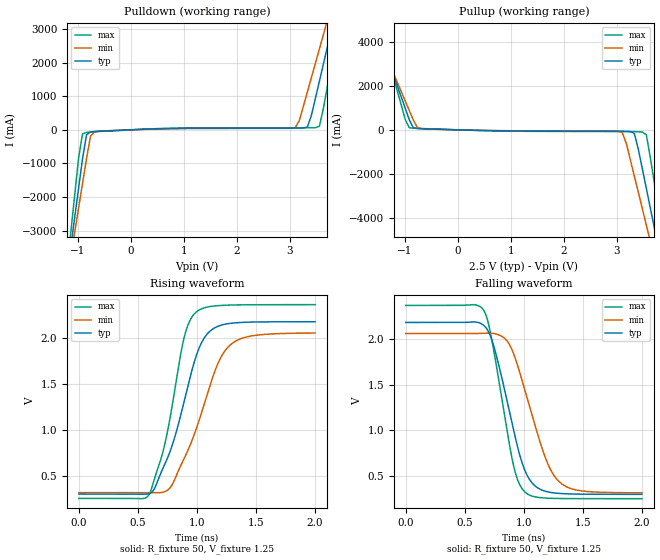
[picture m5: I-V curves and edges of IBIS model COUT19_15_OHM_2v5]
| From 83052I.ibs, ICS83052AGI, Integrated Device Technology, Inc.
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[Model] COUT19_15_OHM_2v5
Model_type   Output
Polarity   Non-Inverting
|   typ   min   max
C_comp   2pF   1.5pF   2.5pF
Vmeas = 1.25V
Rref = 50
Cref = 0
Vref = 1.25V
|   typ   min   max
[Voltage range]   2.5V   2.375V   2.625V
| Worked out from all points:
|   slope of the pulldown table from 0 to 0.375 V, typ, clamps not added: 15.7 ohm
|   slope of the pullup table from 0 to 0.375 V, typ, clamps not added: 15.8 ohm
|   rising waveform, R_fixture 50, V_fixture 1.25: 20-80 % time 248ps typ, 290ps min, 187ps max; typ from 0.303 V to 2.18 V
|   falling waveform, R_fixture 50, V_fixture 1.25: 20-80 % time 207ps typ, 246ps min, 167ps max; typ from 2.18 V to 0.303 V
[Pulldown]
|Voltage   I (typ)   I (min)   I (max)
-2.5V     -19.68A    -17.28A    -23.73A
-1.136V   -3.555A    -3.843A    -3.154A
-1.061V   -2.659A    -3.096A    -2.01A
-909.1mV  -868mA     -1.604A    -120mA
-833.3mV  -148.1mA   -858.1mA   -77.34mA
-681.8mV  -50.66mA   -56.35mA   -57.61mA
3.106V    52.04mA    68.32mA    60.73mA
3.333V    85.78mA    1.134A     61.18mA
3.561V    1.46A      2.417A     111.2mA
3.788V    3A         3.702A     1.969A
3.939V    4.028A     4.56A      3.281A
5V        11.25A     10.58A     12.5A
[Pullup]
|Voltage   I (typ)   I (min)   I (max)
-2.5V     11.3A      9.92A      13.64A
-1.591V   5.096A     4.743A     5.725A
-1.515V   4.579A     4.312A     5.065A
-909.1mV  448.1mA    867.6mA    94.14mA
-681.8mV  51.64mA    49.67mA    60.59mA
3.106V    -66.9mA    -121.9mA   -76.64mA
3.333V    -162.2mA   -2.097A    -82.76mA
3.485V    -1.773A    -3.586A    -98.83mA
3.561V    -2.667A    -4.331A    -227mA
3.712V    -4.455A    -5.822A    -2.419A
3.864V    -6.244A    -7.313A    -4.704A
5V        -19.67A    -18.5A     -21.84A
[Ramp]
|   typ   min   max
dV/dt_r   1.501/0.375n   1.391/0.427n   1.689/0.287n
dV/dt_f   1.505/0.309n   1.394/0.366n   1.693/0.244n
R_load =   50.0000
[Rising Waveform]
R_fixture = 50
V_fixture = 1.25   |Vcc_typ
V_fixture_min = 1.1875 |Vcc_min
V_fixture_max = 1.3125 |Vcc_max
C_fixture = 0.0p
| Time   typ   min   max
0s        302.6mV    318.6mV    255.3mV
592.6ps   305.2mV    318.9mV    293.8mV
706.7ps   568.7mV    321.2mV    738.7mV
776.8ps   782.6mV    377.9mV    1.165V
892.9ps   1.32V      694.1mV    2.014V
995ps     1.813V     1.017V     2.286V
1.071ns   2.02V      1.322V     2.334V
1.169ns   2.125V     1.699V     2.353V
1.291ns   2.162V     1.936V     2.361V
2ns       2.178V     2.056V     2.365V
[Falling Waveform]
R_fixture = 50
V_fixture = 1.25   |Vcc_typ
V_fixture_min = 1.1875 |Vcc_min
V_fixture_max = 1.3125 |Vcc_max
C_fixture = 0.0p
| Time   typ   min   max
0s        2.179V     2.057V     2.365V
660.7ps   2.146V     2.062V     2.311V
698.7ps   2.083V     2.062V     2.174V
748.7ps   1.905V     2.057V     1.847V
846.8ps   1.387V     1.993V     1.084V
912.9ps   1.006V     1.838V     615.7mV
1.017ns   539.5mV    1.402V     319.4mV
1.187ns   334.4mV    685.1mV    261.7mV
1.309ns   311.9mV    429.2mV    257.1mV
2ns       302.7mV    319.4mV    255.3mV
